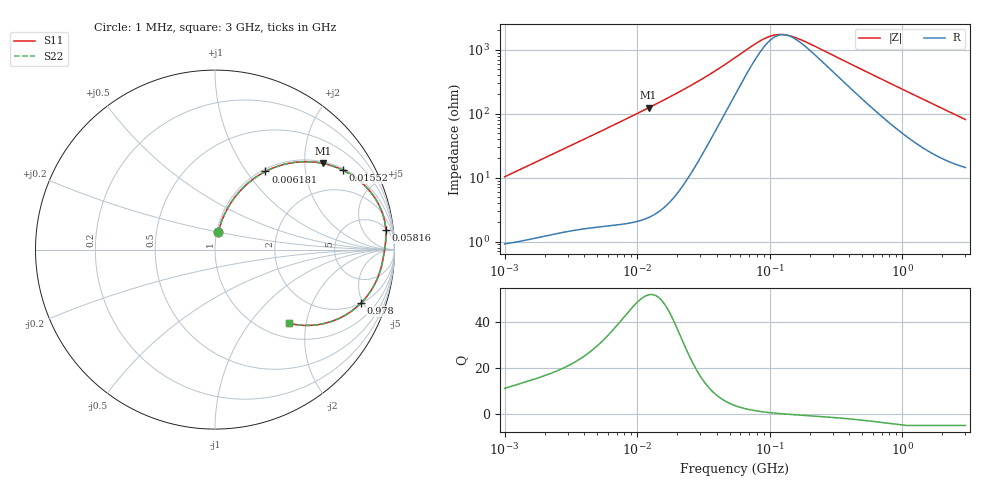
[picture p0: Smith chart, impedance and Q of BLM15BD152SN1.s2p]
! BLM15BD152SN1
# Hz S RI R 50
!Freq.(Hz) S11(Real) S11(Imag) S21(Real) S21(Imag) S12(Real) S12(Imag) S22(Real) S22(Imag)
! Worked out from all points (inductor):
!   401 points, 1 MHz to 3 GHz, reference 50 ohm
!   read as one part in series: L = 1.62 uH near 1.041 MHz
!   highest Q = 52 at 12.21 MHz (marker M1), where L = 1.61 uH
!   self-resonance near 130.6 MHz
!   S11 on the Smith chart (normalised r, x): 1 MHz: 1.02, +0.20; 6.181 MHz: 1.04, +1.23; 15.52 MHz: 1.06, +3.18; 58.16 MHz: 6, +16; 978 MHz: 2.03, -4.84; 3 GHz: 1.29, -1.59
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1000000  0.0192 0.0996  0.9808 -0.0996  0.9808 -0.0996  0.0192 0.0996
2182827  0.0572 0.2055  0.9428 -0.2055  0.9428 -0.2055  0.0572 0.2055
3823119  0.1376 0.3247  0.8624 -0.3247  0.8624 -0.3247  0.1376 0.3247
6180806  0.281 0.4354  0.719 -0.4354  0.719 -0.4354  0.281 0.4354
8861669  0.4416 0.4857  0.5584 -0.4857  0.5584 -0.4857  0.4416 0.4857
1.220676e7  0.6015 0.4801  0.3985 -0.4801  0.3985 -0.4801  0.6015 0.4801
1.461624e7  0.6864 0.4542  0.3136 -0.4542  0.3136 -0.4542  0.6864 0.4542
1.55208e7  0.7126 0.4425  0.2874 -0.4425  0.2874 -0.4425  0.7126 0.4425
2.095589e7  0.8229 0.3676  0.1771 -0.3676  0.1771 -0.3676  0.8229 0.3676
2.773354e7  0.8916 0.2866  0.1084 -0.2866  0.1084 -0.2866  0.8916 0.2866
5.477226e7  0.9513 0.1183  0.0487 -0.1183  0.0487 -0.1183  0.9513 0.1183
5.816196e7  0.9522 0.107  0.0478 -0.107  0.0478 -0.107  0.9522 0.107
8.679508e7  0.9507 0.0459  0.0493 -0.0459  0.0493 -0.0459  0.9507 0.0459
1.125904e8  0.947 0.0155  0.053 -0.0155  0.053 -0.0155  0.947 0.0155
1.460522e8  0.943 -0.0113  0.057 0.0113  0.057 0.0113  0.943 -0.0113
2.094008e8  0.937 -0.0477  0.063 0.0477  0.063 0.0477  0.937 -0.0477
4.66327e8  0.9088 -0.1512  0.0912 0.1512  0.0912 0.1512  0.9088 -0.1512
8.005644e8  0.8516 -0.2538  0.1484 0.2538  0.1484 0.2538  0.8516 -0.2538
9.779672e8  0.814 -0.2972  0.186 0.2972  0.186 0.2972  0.814 -0.2972
1.320433e9  0.7348 -0.36  0.2652 0.36  0.2652 0.36  0.7348 -0.36
1.818868e9  0.6197 -0.409  0.3803 0.409  0.3803 0.409  0.6197 -0.409
3e9  0.4113 -0.4101  0.5887 0.4101  0.5887 0.4101  0.4113 -0.4101
